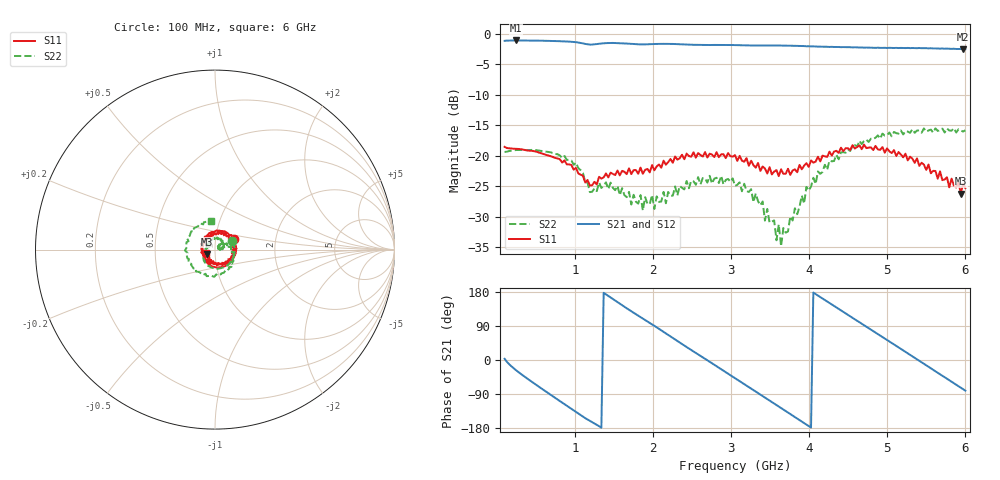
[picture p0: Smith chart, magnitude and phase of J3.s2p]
!Agilent Technologies,E8364B,MY43040379,A.07.50.67
!Agilent E8364B: A.07.50.67
!Date: Tuesday, March 24, 2026 11:37:10
!Correction: S11(Full 2 Port(1,2))
!S21(Full 2 Port(1,2))
!S12(Full 2 Port(1,2))
!S22(Full 2 Port(1,2))
!S2P File: Measurements: S11, S21, S12, S22:
# Hz S  dB  R 50
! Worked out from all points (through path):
!   201 points, 100 MHz to 6 GHz, reference 50 ohm
!   highest |S21| = -1.12 dB at 247.5 MHz (marker M1); lowest = -2.5 dB at 5.971 GHz (marker M2)
!   group delay of S21, straight-line fit = 372 ps
!   lowest |S11| = -26.2 dB at 5.941 GHz (marker M3), VSWR 1.10, Z = 45.9 - j2.24 ohm
!   |S11| at or under -10 dB: start of sweep to end of sweep
!   |S22| runs from -34.8 to -15.5 dB; largest |S21 - S12| = 0.0024
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1e8  -18.53 29.2  -1.18 3.1  -1.18 3.1  -19.37 25.4
2.475e8  -18.86 -15.1  -1.12 -27.1  -1.12 -27.2  -19.06 -16.4
6.605e8  -19.96 -81.7  -1.18 -87.8  -1.18 -87.9  -19.36 -81.8
1.103e9  -23.26 -149.5  -1.59 -149.7  -1.59 -149.8  -22.82 -153.7
1.1915e9  -24.88 -156.6  -1.79 -160.4  -1.79 -160.5  -25.95 -159.5
1.516e9  -23.15 173.1  -1.54 156.8  -1.53 156.7  -25.64 -176.6
1.7815e9  -22.35 130.6  -1.74 120.9  -1.74 120.8  -27.53 155.5
2.0765e9  -21.43 98.0  -1.68 82.2  -1.68 82.1  -27.55 139.8
2.578e9  -19.55 37.4  -1.86 14.8  -1.86 14.7  -23.49 96.0
3.05e9  -19.89 -32.7  -1.87 -48.1  -1.86 -48.2  -24.94 39.0
3.345e9  -21.17 -82.0  -1.95 -87.3  -1.94 -87.3  -27.44 4.9
3.5515e9  -22.58 -121.1  -1.93 -114.8  -1.94 -114.8  -30.58 -0.9
3.581e9  -22.35 -135.5  -1.94 -118.8  -1.94 -118.9  -33.85 22.6
3.6105e9  -23.34 -139.2  -1.94 -122.8  -1.94 -122.8  -31.24 18.6
3.64e9  -22.21 -143.2  -1.95 -126.8  -1.94 -126.8  -34.80 11.4
4.053e9  -21.12 117.5  -2.08 177.9  -2.09 177.9  -23.60 29.5
4.584e9  -18.81 35.0  -2.23 107.4  -2.24 107.5  -18.24 -39.9
5.0265e9  -19.27 -23.5  -2.32 49.0  -2.33 49.0  -16.19 -107.4
5.469e9  -21.46 -79.4  -2.38 -10.0  -2.38 -10.1  -15.53 -178.5
5.941e9  -26.18 -150.2  -2.51 -73.1  -2.52 -73.1  -15.84 103.9
5.9705e9  -24.63 -147.9  -2.55 -77.0  -2.54 -76.9  -16.03 103.1
6e9  -25.29 -158.2  -2.53 -80.9  -2.53 -80.9  -15.83 97.5
